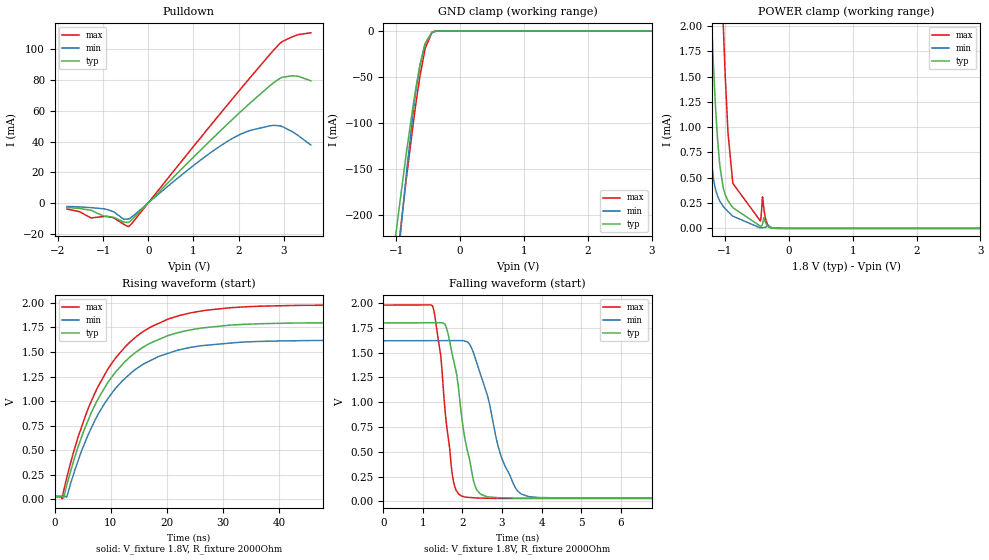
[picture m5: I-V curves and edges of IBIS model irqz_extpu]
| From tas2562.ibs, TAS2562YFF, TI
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|   irqz_extpu Model
[Model]   irqz_extpu
Model_type   Open_drain
Polarity   Non-Inverting
Vmeas = 0.9
Vref = 1.8
Cref = 2pF
Rref = 2000
|   typ   min   max
C_comp   2.003pF   1.966pF   2.088pF
| Where Nom  PVT is Nominal Process, 1.8V, 25C
|   Fast PVT is Strong Process,  1.98V, -40C
|   Slow PVT is Weak Process,   1.62V, 150C
[Voltage Range]   1.8   1.62   1.98
|Junction Temperature
[Temperature Range]   25   150   -40
[Pullup Reference]   1.8   1.62   1.98
[Pulldown Reference]   0   0   0
[Power Clamp Reference]   1.8   1.62   1.98
[GND Clamp Reference]   0   0   0
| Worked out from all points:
|   slope of the pulldown table from 0 to 0.27 V, typ, clamps not added: 33.2 ohm
|   GND clamp passes 1 mA (typ) near -0.43 V on its own axis
|   POWER clamp passes 1 mA (typ) near -1.13 V on its own axis
|   falling waveform, V_fixture 1.8V, R_fixture 2000Ohm: 20-80 % time 436ps typ, 647ps min, 299ps max; typ from 1.8 V to 0.029 V
|   rising waveform, V_fixture 1.8V, R_fixture 2000Ohm: 20-80 % time 10ns typ, 10ns min, 10.1ns max; typ from 0.029 V to 1.8 V
[Pulldown]
|   Voltage   I(typ)   I(min)   I(max)
-1.8V     -2.957mA   -2.3mA     -4.034mA
-1.525V   -3.634mA   -2.61mA    -5.679mA
-1.26V    -4.892mA   -3.1mA     -9.788mA
-925.2mV  -8.723mA   -4.215mA   -8.896mA
-547.2mV  -12.42mA   -10.54mA   -13.89mA
-412.2mV  -12.21mA   -10.16mA   -14.9mA
1.246V    36.9mA     29.82mA    45.63mA
2.137V    61.88mA    45.94mA    77.46mA
2.693V    76.31mA    50.21mA    96.73mA
2.957V    81.7mA     49.87mA    104.9mA
3.276V    82.66mA    44.75mA    109.2mA
3.6V      79.58mA    37.74mA    110.8mA
[GND Clamp]
|   Voltage   I(typ)   I(min)   I(max)
-1.8V     -830.2mA   -917.2mA   -810.3mA
-1.017V   -226mA     -280.9mA   -265mA
-849.6mV  -136.2mA   -160.2mA   -164.9mA
-725.4mV  -76.2mA    -82.49mA   -95.68mA
-676.8mV  -55.51mA   -57.51mA   -71.17mA
-628.2mV  -37.22mA   -36.99mA   -48.97mA
-558mV    -16.53mA   -16.23mA   -22.83mA
-541.8mV  -12.94mA   -12.9mA    -18.1mA
-439.2mV  -1.277mA   -1.972mA   -1.711mA
-385.2mV  -225.2uA   -567.9uA   -219.6uA
-261mV    -2.196uA   -22.38uA   -650.9nA
3.6V      0A         0A         0A
[POWER Clamp]
|   Voltage   I(typ)   I(min)   I(max)
-1.8V     15.69mA    11.82mA    24.27mA
-1.352V   4.592mA    2.132mA    9.4mA
-1.249V   2.667mA    900.4uA    6.926mA
-1.152V   1.249mA    396.7uA    4.653mA
-1.082V   632.3uA    271.2uA    3.097mA
-1.022V   390.1uA    214.6uA    1.943mA
-952.2mV  272.5uA    165.5uA    941.7uA
-876.6mV  204.9uA    120.4uA    444.5uA
-444.6mV  21.3uA     4.377uA    72.73uA
-412.2mV  43.5uA     7.407uA    311.6uA
-261mV    1.982uA    6.997uA    3.314uA
3.6V      0A         0A         0A
[Ramp]
R_load = 2000
|   typ   min   max
dV/dt_r   1.06242/1.00173e-08   0.953166/1.00375e-08   1.17202/1.01512e-08
dV/dt_f   1.06242/4.37123e-10   0.953167/6.50629e-10   1.17202/2.98021e-10
[Falling Waveform]
V_fixture = 1.8V
V_fixture_min = 1.62V
V_fixture_max = 1.98V
R_fixture = 2000Ohm
C_fixture = 0F
|   Time   V(typ)   V(min)   V(max)
0s        1.8V       1.62V      1.98V
1.242ns   1.801V     1.621V     1.97V
1.446ns   1.801V     1.621V     1.478V
1.557ns   1.785V     1.621V     924.3mV
1.773ns   1.425V     1.621V     197.3mV
2.083ns   584.9mV    1.613V     41.93mV
2.454ns   72.03mV    1.283V     32.66mV
2.99ns    35.53mV    438.9mV    28.29mV
3.714ns   31.24mV    45.18mV    28.28mV
50ns      29.3mV     31.34mV    26.38mV
[Rising Waveform]
V_fixture = 1.8V
V_fixture_min = 1.62V
V_fixture_max = 1.98V
R_fixture = 2000Ohm
C_fixture = 0F
|   Time   V(typ)   V(min)   V(max)
0s        29.3mV     31.34mV    26.38mV
1.277ns   29.26mV    31.35mV    6.36mV
1.578ns   13.25mV    31.35mV    82.93mV
2.123ns   139.4mV    22.42mV    215.4mV
4.194ns   540.6mV    399.1mV    640.3mV
7.12ns    955mV      798.8mV    1.079V
12.5ns    1.401V     1.23V      1.55V
20.25ns   1.668V     1.488V     1.837V
31.21ns   1.774V     1.591V     1.951V
500ns     1.8V       1.62V      1.98V
